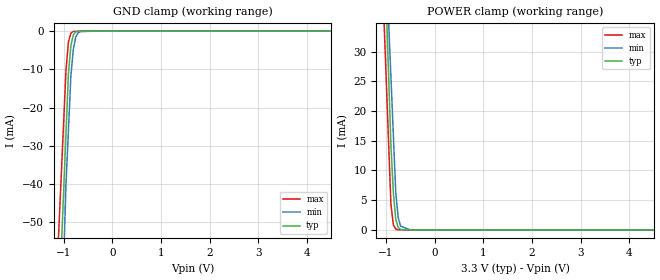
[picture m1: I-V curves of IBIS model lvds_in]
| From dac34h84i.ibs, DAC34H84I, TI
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[Model] lvds_in
Model_type Input
Vinl = 1.12500V
Vinh = 1.27500V
C_comp 892.000fF 876.000fF 908.000fF
| variable typ   min   max
[Voltage Range] 3.30000V 3.00000V 3.60000V
[POWER Clamp Reference] 3.30000V 3.00000V 3.60000V
[GND Clamp Reference] 0.00000V 0.00000V 0.00000V
[Temperature Range] 25   125   -40
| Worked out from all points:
|   GND clamp passes 1 mA (typ) near -0.80 V on its own axis
|   POWER clamp passes 1 mA (typ) near -0.77 V on its own axis
[GND Clamp]
-3.3V     -762.6mA   -1.019A    -676.4mA
-950mV    -26.8mA    -40.05mA   -10.23mA
-900mV    -11.14mA   -25.96mA   -2.842mA
-850mV    -3.845mA   -11.86mA   -548.1uA
-800mV    -995.9uA   -4.821mA   -82.69uA
-750mV    -210.4uA   -1.54mA    -72.49uA
-700mV    -38.09uA   -425.1uA   -62.29uA
-650mV    -32.93uA   -116.5uA   -52.09uA
-400mV    -7.114uA   -31.3uA    -1.107uA
-350mV    -1.951uA   -14.26uA   -1.081uA
-325mV    -1.928uA   -5.733uA   -1.069uA
6.6V      4.441uA    10.15uA    2.424uA
[POWER Clamp]
-3.3V     606.8mA    494.2mA    526.1mA
-1.05V    51.29mA    55mA       36.92mA
-900mV    14.25mA    25.72mA    4.307mA
-850mV    6.252mA    15.96mA    865.9uA
-800mV    1.759mA    6.195mA    140.3uA
-750mV    391.1uA    2.046mA    16.55uA
-700mV    72.45uA    636uA      14.97uA
-500mV    31.05uA    10.52uA    8.669uA
6.6V      0A         0A         0A
